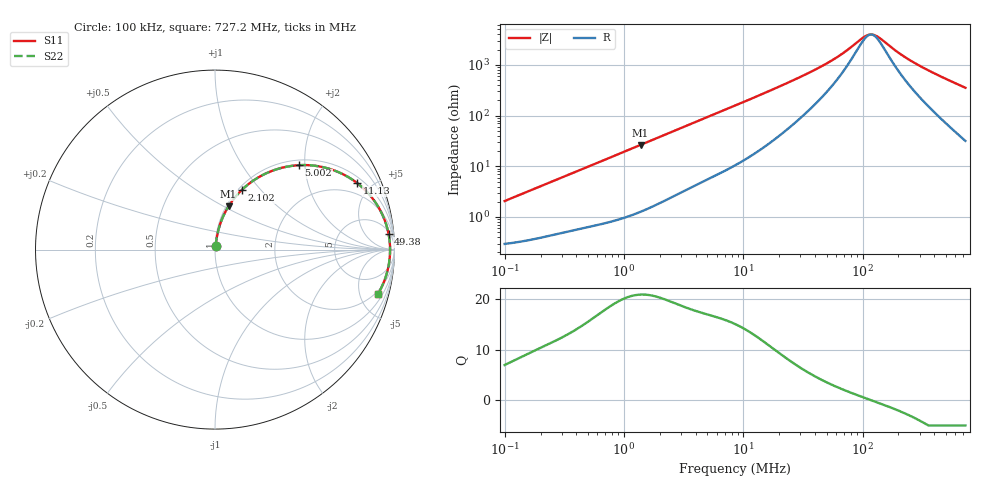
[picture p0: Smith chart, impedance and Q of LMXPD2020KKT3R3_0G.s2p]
! LMXPD2020KKT3R3_0G  S-PARAMETER MODEL  ( General Type )
! Model Generated by TAIYO YUDEN Corporation (http://www.ty-top.com)
! Version 1.0
! TAIYO YUDEN Control No. 191023NI43SB-FBB
! Copyright(c) 2019 TAIYO YUDEN CO.,LTD. All Rights Reserved.
! Product Description (link to TY-COMPAS)
! https://ds.yuden.co.jp/TYCOMPAS/or/detail?pn=LMXPD2020KKT3R3M0G&u=M
! Products Name : Inductors
! Characteristics :
!  Inductance : 3.3 uH , SRF(min) : -Hz , DC Resistance(max) : 0.3 Ohm
!  Rated Current : Saturation :880 mA , Temp Rise : 1000 mA
!  Case Size : 2.0 x 2.0 / 0.079 x 0.079 [mm/inch] , Thickness : 1 / 0.039 [mm/inch]
!  (Conditions: Temperature = 25 degC , DC Bias Current/Voltage = 0A / 0V)
! External Node Assignments :
!  1  o---GGG---o  2
! GND o---------o GND
! Frequency Range : 0.1MHz  -  727.209926MHz  [ 402 STEP ]
# MHz S RI R 50
! Freq[MHz].  S11 Real  S11 Imag  S21 Real  S21 Imag  S12 Real  S12 Imag  S22 Real  S22 Imag
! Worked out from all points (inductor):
!   401 points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, 100 kHz to 727.2 MHz, reference 50 ohm
!   read as one part in series: L = 3.25 uH near 104.5 kHz
!   highest Q = 20.9 at 1.378 MHz (marker M1), where L = 3.06 uH
!   self-resonance near 117.8 MHz
!   S11 on the Smith chart (normalised r, x): 100 kHz: 1.01, +0.04; 2.102 MHz: 1.04, +0.80; 5.002 MHz: 1.11, +1.86; 11.13 MHz: 1.30, +4.09; 49.38 MHz: 7, +20; 727.2 MHz: 1.63, -7.06
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0.1  0.00336 0.0203  0.9966 -0.0203  0.9966 -0.0203  0.00336 0.0203
0.443433  0.0133 0.0855  0.9867 -0.0855  0.9867 -0.0855  0.0133 0.0855
0.79038  0.0305 0.1474  0.9695 -0.1474  0.9695 -0.1474  0.0305 0.1474
1.377811  0.0757 0.2416  0.9243 -0.2416  0.9243 -0.2416  0.0757 0.2416
1.966328  0.1355 0.3185  0.8645 -0.3185  0.8645 -0.3185  0.1355 0.3185
2.101931  0.1506 0.3336  0.8494 -0.3336  0.8494 -0.3336  0.1506 0.3336
3.136124  0.2706 0.4181  0.7294 -0.4181  0.7294 -0.4181  0.2706 0.4181
5.001846  0.4669 0.4703  0.5331 -0.4703  0.5331 -0.4703  0.4669 0.4703
8.719349  0.7087 0.4221  0.2913 -0.4221  0.2913 -0.4221  0.7087 0.4221
11.13473  0.7913 0.3712  0.2087 -0.3712  0.2087 -0.3712  0.7913 0.3712
18.98363  0.9042 0.2472  0.0958 -0.2472  0.0958 -0.2472  0.9042 0.2472
37.81446  0.9592 0.1218  0.0408 -0.1218  0.0408 -0.1218  0.9592 0.1218
49.37507  0.9673 0.0865  0.0327 -0.0865  0.0327 -0.0865  0.9673 0.0865
68.91598  0.9728 0.0498  0.0272 -0.0498  0.0272 -0.0498  0.9728 0.0498
100.5635  0.9753 0.0141  0.0247 -0.0141  0.0247 -0.0141  0.9753 0.0141
112.3857  0.9755 0.00415  0.0245 -0.00415  0.0245 -0.00415  0.9755 0.00415
120.1361  0.9755 -0.00178  0.0245 0.00178  0.0245 0.00178  0.9755 -0.00178
131.3077  0.9754 -0.0097  0.0246 0.0097  0.0246 0.0097  0.9754 -0.0097
167.6818  0.9745 -0.032  0.0255 0.032  0.0255 0.032  0.9745 -0.032
223.8669  0.9718 -0.0609  0.0282 0.0609  0.0282 0.0609  0.9718 -0.0609
305.5962  0.9658 -0.0972  0.0342 0.0972  0.0342 0.0972  0.9658 -0.0972
727.2099  0.9073 -0.2485  0.0927 0.2485  0.0927 0.2485  0.9073 -0.2485
